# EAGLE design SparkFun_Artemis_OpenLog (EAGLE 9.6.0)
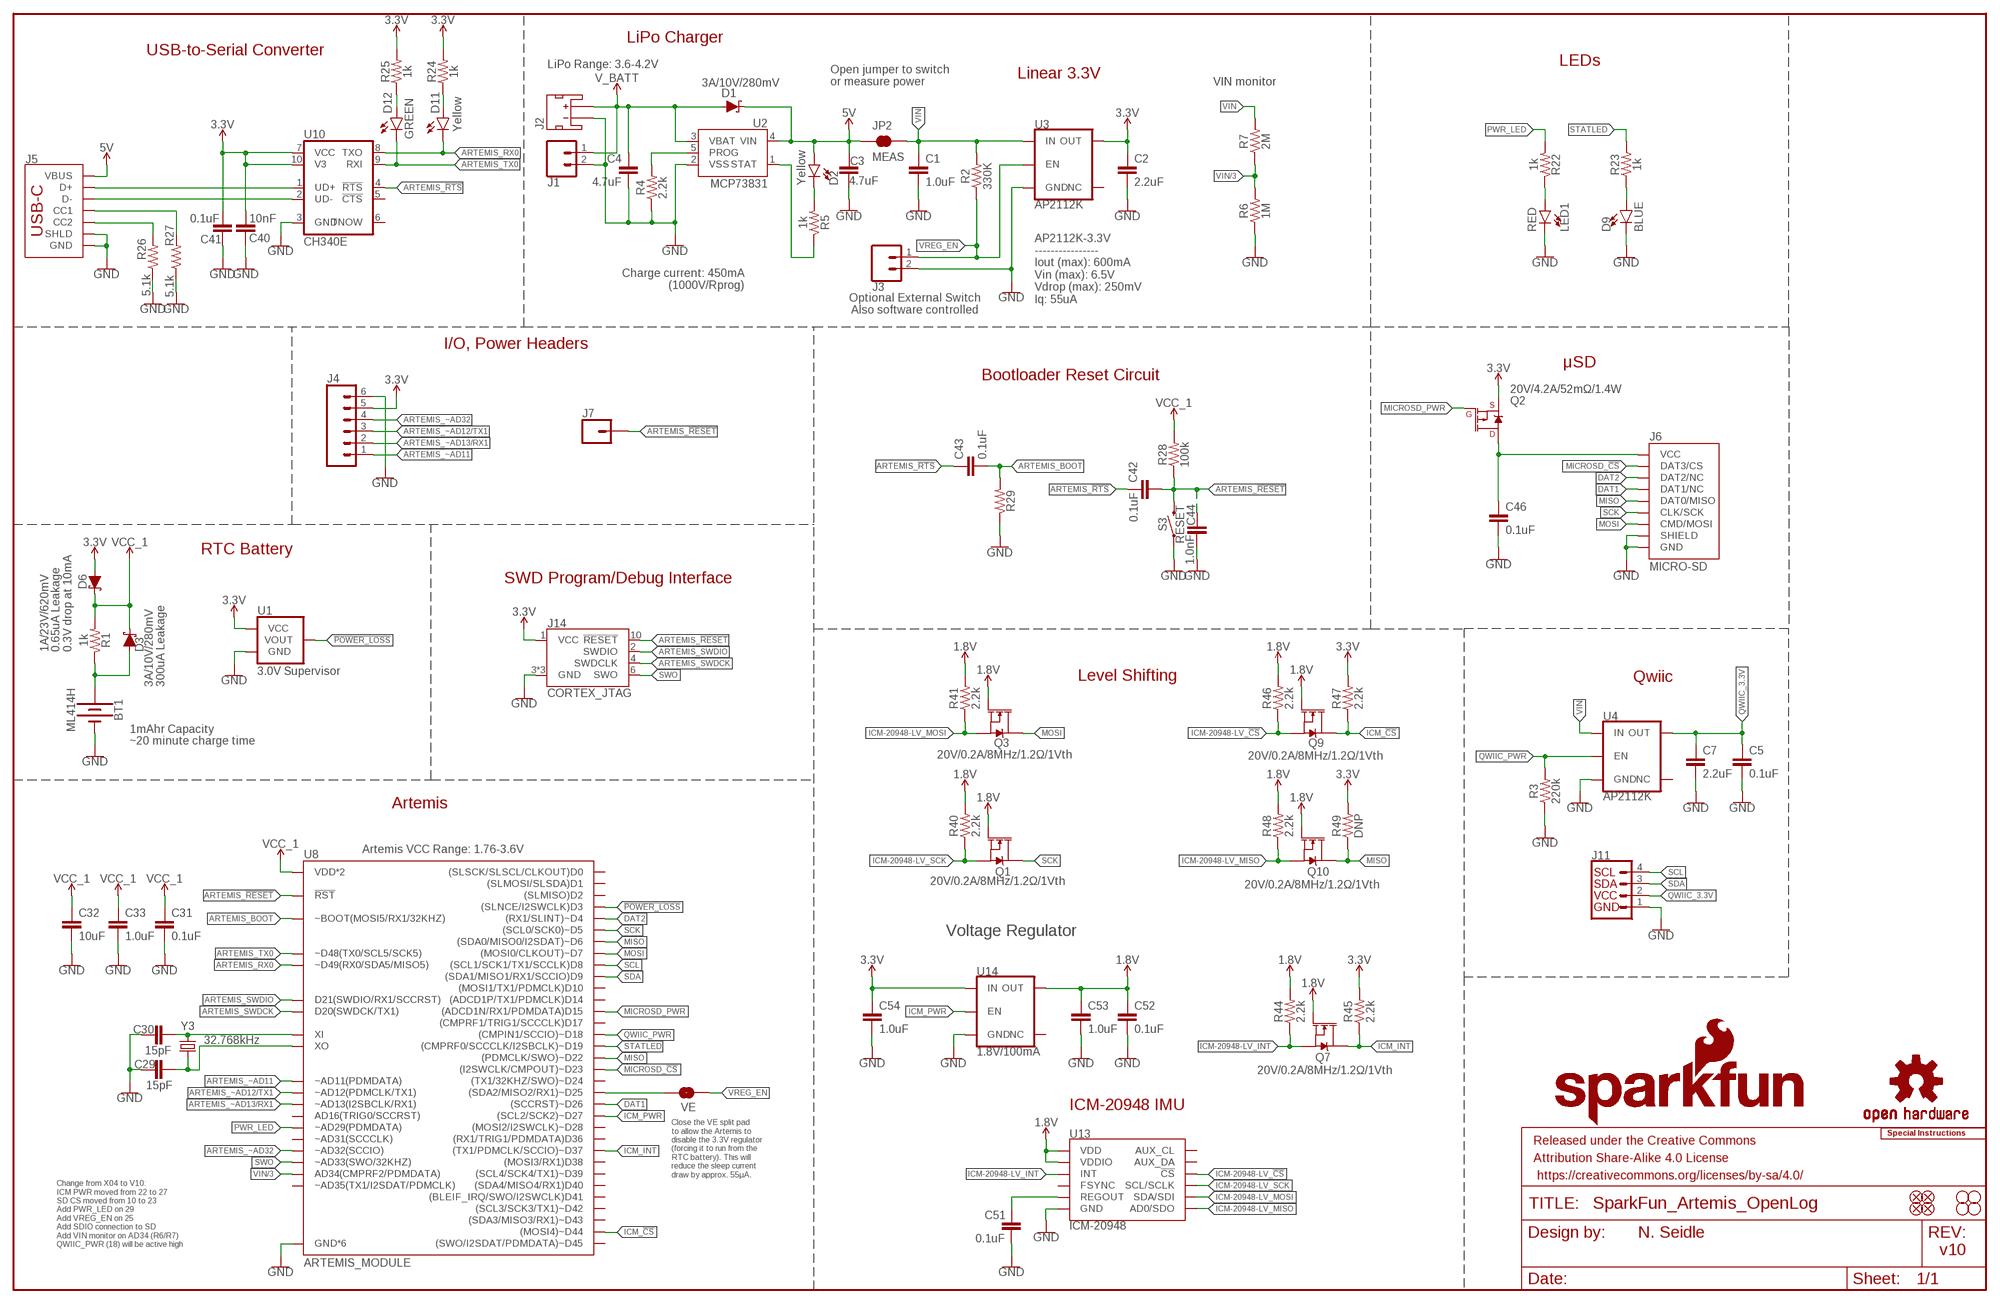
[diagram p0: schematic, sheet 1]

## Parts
BT1  ML414H  ML414H_IV01E_BATTERY  [ML414H_IV01E]
C1  1.0uF  1.0UF-0402T-16V-10%  [0402-TIGHT]
C2  2.2uF  2.2UF-0402_TIGHT-10V-10%-X5R  [0402-TIGHT]
C3  4.7uF  4.7UF-0402_TIGHT-6.3V-20%-X5R  [0402-TIGHT]
C4  4.7uF  4.7UF-0402_TIGHT-6.3V-20%-X5R  [0402-TIGHT]
C5  0.1uF  0.1UF-0402T-6.3V-10%-X7R  [0402-TIGHT]
C7  2.2uF  2.2UF-0402_TIGHT-10V-10%-X5R  [0402-TIGHT]
C29  15pF  15PF-0402T-50V-5%  [0402-TIGHT]
C30  15pF  15PF-0402T-50V-5%  [0402-TIGHT]
C31  0.1uF  0.1UF-0402T-16V-10%  [0402-TIGHT]
C32  10uF  10UF-0402T-6.3V-20%  [0402-TIGHT]
C33  1.0uF  1.0UF-0402T-16V-10%  [0402-TIGHT]
C40  10nF  10NF-0402T-25V-10%  [0402-TIGHT]
C41  0.1uF  0.1UF-0402T-16V-10%  [0402-TIGHT]
C42  0.1uF  0.1UF-0402T-16V-10%  [0402-TIGHT]
C43  0.1uF  0.1UF-0402T-16V-10%  [0402-TIGHT]
C44  1.0nF  1.0NF/1000PF-0402_TIGHT-50V-10%  [0402-TIGHT]
C46  0.1uF  0.1UF-0402T-16V-10%  [0402-TIGHT]
C51  0.1uF  0.1UF-0402T-16V-10%  [0402-TIGHT]
C52  0.1uF  0.1UF-0402T-16V-10%  [0402-TIGHT]
C53  1.0uF  1.0UF-0402T-16V-10%  [0402-TIGHT]
C54  1.0uF  1.0UF-0402T-16V-10%  [0402-TIGHT]
D1  3A/10V/280mV  DIODE-SCHOTTKY-BAT60A  [SOD-323]
D2  Yellow  LED-YELLOW0603  [LED-0603]
D3  3A/10V/280mV  DIODE-SCHOTTKY-BAT60A  [SOD-323]
D6  1A/23V/620mV  DIODE-SCHOTTKY-BAT20J  [SOD-323]
D9  BLUE  LED-BLUE0603  [LED-0603]
D11  Yellow  LED-YELLOW0603  [LED-0603]
D12  GREEN  LED-GREEN0603  [LED-0603]
FD1  FIDUCIAL1X2  [FIDUCIAL-1X2]
FD2  FIDUCIAL1X2  [FIDUCIAL-1X2]
FD3  FIDUCIAL1X2  [FIDUCIAL-1X2]
FD4  FIDUCIAL1X2  [FIDUCIAL-1X2]
FRAME1  FRAME-LEDGER  [CREATIVE_COMMONS]
H1  STAND-OFF  [STAND-OFF]
H2  STAND-OFF  [STAND-OFF]
H3  STAND-OFF  [STAND-OFF]
H4  STAND-OFF  [STAND-OFF]
J1  CONN_021X02_NO_SILK  [1X02_NO_SILK]
J2  JST_2MM_MALE  [JST-2-SMD]
J3  CONN_021X02_NO_SILK  [1X02_NO_SILK]
J4  CONN_06NO_SILK_NO_POP  [1X06_NO_SILK]
J5  USB_C_4-LAYER_PADS  [USB-C-16P_4LAYER-PADS]
J6  MICRO-SD  MICRO-SD-SDIOPUSH-PUSH  [MICRO-SD-SOCKET]
J7  CONN_01PTH_NO_SILK_YES_STOP  [1X01_NO_SILK]
J11  QWIIC_CONNECTORJS-1MM  [JST04_1MM_RA]
J14  CORTEX_JTAG  CORTEX_JTAG_DEBUG_MINIMUM_PTH  [2X5-PTH-1.27MM]
JP2  MEAS  JUMPER-COMBO_2_NC_TRACE  [COMBO-JUMPER_2_NC_TRACE]
LED1  RED  LED-RED0603  [LED-0603]
LOGO1  SFE_LOGO_NAME.1_INCH  [SFE_LOGO_NAME_.1]
LOGO2  OSHW-LOGOS  [OSHW-LOGO-S]
LOGO3  SPECIAL_INSTRUCTIONS-ORDERING  [ORDERING_INSTRUCTIONS]
LOGO4  SFE_LOGO_FLAME.1_INCH  [SFE_LOGO_FLAME_.1]
LOGO5  SFE_LOGO_FLAME.1_INCH  [SFE_LOGO_FLAME_.1]
Q1  20V/0.2A/8MHz/1.2Ω/1Vth  MOSFET-NCH-RE1C00UNTL  [SOT-416FL]
Q2  20V/4.2A/52mΩ/1.4W  MOSFET_PCH-DMG2305UX-7  [SOT23-3]
Q3  20V/0.2A/8MHz/1.2Ω/1Vth  MOSFET-NCH-RE1C00UNTL  [SOT-416FL]
Q7  20V/0.2A/8MHz/1.2Ω/1Vth  MOSFET-NCH-RE1C00UNTL  [SOT-416FL]
Q9  20V/0.2A/8MHz/1.2Ω/1Vth  MOSFET-NCH-RE1C00UNTL  [SOT-416FL]
Q10  20V/0.2A/8MHz/1.2Ω/1Vth  MOSFET-NCH-RE1C00UNTL  [SOT-416FL]
R1  1k  1KOHM-0402T-1/16W-1%  [0402-TIGHT]
R2  330K  330KOHM-0402T-1/16W-1%  [0402-TIGHT]
R3  220k  220KOHM-0402T-1/16W-1%  [0402-TIGHT]
R4  2.2k  2.2KOHM-0402T-1/16W-1%  [0402-TIGHT]
R5  1k  1KOHM-0402T-1/16W-1%  [0402-TIGHT]
R6  1M  1MOHM-0402T-1/16W-1%  [0402-TIGHT]
R7  2M  2MOHM-0402T-1/16W-1%  [0402-TIGHT]
R22  1k  1KOHM-0402T-1/16W-1%  [0402-TIGHT]
R23  1k  1KOHM-0402T-1/16W-1%  [0402-TIGHT]
R24  1k  1KOHM-0402T-1/16W-1%  [0402-TIGHT]
R25  1k  1KOHM-0402T-1/16W-1%  [0402-TIGHT]
R26  5.1k  5.1KOHM-0402T-1/16W-1%  [0402-TIGHT]
R27  5.1k  5.1KOHM-0402T-1/16W-1%  [0402-TIGHT]
R28  100k  100KOHM-0402T-1/16W-1%  [0402-TIGHT]
R29  220KOHM-0402T-1/16W-1%  [0402-TIGHT]
R40  2.2k  2.2KOHM-0402T-1/16W-1%  [0402-TIGHT]
R41  2.2k  2.2KOHM-0402T-1/16W-1%  [0402-TIGHT]
R44  2.2k  2.2KOHM-0402T-1/16W-1%  [0402-TIGHT]
R45  2.2k  2.2KOHM-0402T-1/16W-1%  [0402-TIGHT]
R46  2.2k  2.2KOHM-0402T-1/16W-1%  [0402-TIGHT]
R47  2.2k  2.2KOHM-0402T-1/16W-1%  [0402-TIGHT]
R48  2.2k  2.2KOHM-0402T-1/16W-1%  [0402-TIGHT]
R49  DNP  RESISTOR0402T  [0402-TIGHT]
S3  RESET  MOMENTARY-SWITCH-SPST-SMD-4.6X2.8MM  [TACTILE_SWITCH_SMD_4.6X2.8MM]
U1  3.0V Supervisor  V_SUPERVISOR  [SOT23-3]
U2  MCP73831  [SOT23-5]
U3  AP2112K  V_REG_AP2112K-3.3V  [SOT23-5]
U4  AP2112K  V_REG_AP2112K-3.3V  [SOT23-5]
U8  ARTEMIS_MODULE  ARTEMIS_MODULESMD  [ARTEMIS_FP]
U10  CH340E  CH340E_MSOP10  [MSOP10]
U13  ICM-20948  [QFN24-3X3]
U14  1.8V/100mA  V_REG_SP6214-1.8V  [SC70]
VE  JUMPER-SMT_2_NO_SILK  [SMT-JUMPER_2_NO_SILK]
Y3  32.768kHz  CRYSTAL-32.768KHZSMD-3.2X1.5  [CRYSTAL-SMD-3.2X1.5MM]

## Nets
3.3V: C2.1 C40.1 C41.1 C54.1 D6.A J4.5 J14.1(VCC) Q2.2(S) R24.2 R25.2 R45.2 R47.2 R49.2 U1.3(VCC) U3.5(OUT) U10.7(VCC) U10.10(V3) U14.1(IN)
5V [Power]: C3.1 D1.C D2.A J5.VBUS1(VBUS) J5.VBUS2(VBUS) JP2.1 JP2.3 U2.4(VIN)
!POWER_LOSS!: U1.2(VOUT) U8.D3((SLNCE/I2SWCLK)D3)
ARTEMIS_!RESET: C42.2 C44.1 J7.1 J14.10(!RESET) R28.1 S3.3 S3.4 U8.~RST(!RST)
ARTEMIS_!RTS!: C42.1 C43.1 U10.4(!RTS)
ARTEMIS_BOOT: C43.2 R29.2 U8.BOOT(~BOOT(MOSI5/RX1/32KHZ))
ARTEMIS_RX0: D11.C U8.RXI-0(~D49(RX0/SDA5/MISO5)) U10.8(TXO)
ARTEMIS_SWDCK: J14.4(SWDCLK) U8.SWDCK(D20(SWDCK/TX1))
ARTEMIS_SWDIO: J14.2(SWDIO) U8.SWDIO(D21(SWDIO/RX1/SCCRST))
ARTEMIS_TX0: D12.C U8.TXO-0(~D48(TX0/SCL5/SCK5)) U10.9(RXI)
ARTEMIS_~AD11: J4.1 U8.~AD11(~AD11(PDMDATA))
ARTEMIS_~AD12/TX1: J4.3 U8.~AD12(~AD12(PDMCLK/TX1))
ARTEMIS_~AD13/RX1: J4.2 U8.~AD13(~AD13(I2SBCLK/RX1))
ARTEMIS_~AD32: J4.4 U8.~AD32(~AD32(SCCIO))
CC3: J5.B5(CC2) R26.2
CC4: J5.A5(CC1) R27.2
CHG_LED: R5.1 U2.1(STAT)
D+2: J5.A6(D+) J5.B6(D+) U10.1(UD+)
D-2: J5.A7(D-) J5.B7(D-) U10.2(UD-)
DAT1: J6.RSV2(DAT1/NC) U8.~D26((SCCRST)~D26)
DAT2: J6.RSV1(DAT2/NC) U8.~D4((RX1/SLINT)~D4)
GND: BT1.- C1.2 C2.2 C3.2 C4.2 C5.2 C7.2 C29.1 C30.1 C31.1 C32.2 C33.2 C40.2 C41.2 C44.2 C46.2 C51.2 C52.2 C53.2 C54.2 D9.C J1.2 J2.1(-) J3.2 J4.6 J5.GND J5.GND2(GND) J5.SHLD1(SHLD) J5.SHLD2(SHLD) J5.SHLD3(SHLD) J5.SHLD4(SHLD) J6.CD1(SHIELD) J6.GND J6.GND1(GND) J6.GND3(GND) J11.1 J14.3(GND) J14.5(GND) J14.9(GND) LED1.C R3.1 R4.1 R6.1 R26.1 R27.1 R29.1 S3.1 S3.2 U1.1(GND) U2.2(VSS) U3.2(GND) U4.2(GND) U8.GND@1(GND*6) U8.GND@22(GND*6) U8.GND@38(GND*6) U8.GND@39(GND*6) U8.GND@47(GND*6) U8.GND@59(GND*6) U10.3(GND) U13.18(GND) U13.20(GND) U14.2(GND)
ICM-20948-LV_!CS!: Q9.2(S) R46.1 U13.22(!CS)
ICM-20948-LV_#_1.8V: C52.1 C53.1 Q1.1(G) Q3.1(G) Q7.1(G) Q9.1(G) Q10.1(G) R40.2 R41.2 R44.2 R46.2 R48.2 U13.8(VDDIO) U13.13(VDD) U14.5(OUT) ; supply symbol labelled 1.8V
ICM-20948-LV_INT: Q7.2(S) R44.1 U13.12(INT)
ICM-20948-LV_MISO: Q10.2(S) R48.1 U13.9(AD0/SDO)
ICM-20948-LV_MOSI: Q3.2(S) R41.1 U13.24(SDA/SDI)
ICM-20948-LV_SCK: Q1.2(S) R40.1 U13.23(SCL/SCLK)
ICM_!CS!: Q9.3(D) R47.1 U8.~D44((MOSI4)~D44)
ICM_INT: Q7.3(D) R45.1 U8.~D37((TX1/PDMCLK/SCCIO)~D37)
ICM_PWR: U8.~D27((SCL2/SCK2)~D27) U14.3(EN)
MICROSD_!CS!: J6.CS(DAT3/CS) U8.~D23((I2SWCLK/CMPOUT)~D23)
MICROSD_PWR: Q2.1(G) U8.D15((ADCD1N/RX1/PDMDATA)D15)
MISO: J6.DO(DAT0/MISO) Q10.3(D) R49.1 U8.~D6((SDA0/MISO0/I2SDAT)~D6) U8.~D22((PDMCLK/SWO)~D22)
MOSI: J6.DI(CMD/MOSI) Q3.3(D) U8.D7((MOSI0/CLKOUT)~D7)
N$1: BT1.+ D3.A R1.1
N$7: R4.2 U2.5(PROG)
N$11: D2.C R5.2
N$20: C29.2 U8.XO Y3.P$2
N$21: C30.2 U8.XI Y3.P$1
N$24: LED1.A R22.1
N$25: D9.A R23.1
N$26: D12.A R25.1
N$27: D11.A R24.1
N$30: C51.1 U13.10(REGOUT)
PWR_LED: R22.2 U8.~AD29(~AD29(PDMDATA))
QWIIC_3.3V: C5.1 C7.1 J11.2 U4.5(OUT)
QWIIC_PWR: R3.2 U4.3(EN) U8.~D18((CMPIN1/SCCIO)~D18)
SCK: J6.SCLK(CLK/SCK) Q1.3(D) U8.~D5((SCL0/SCK0)~D5)
SCL: J11.4 U8.D8((SCL1/SCK1/TX1/SCCLK)D8)
SD_PWR: C46.1 J6.VCC Q2.3(D)
SDA: J11.3 U8.D9((SDA1/MISO1/RX1/SCCIO)D9)
STATLED: R23.2 U8.~D19((CMPRF0/SCCCLK/I2SBCLK)~D19)
SWO: J14.6(SWO) U8.~AD33/SWO(~AD33(SWO/32KHZ))
V_BATT: C4.1 D1.A J1.1 J2.2(+) U2.3(VBAT)
VCC_1: C31.2 C32.1 C33.1 D3.C D6.C R1.2 R28.2 U8.VDD@36(VDD*2) U8.VDD@37(VDD*2)
VIN [Power]: C1.1 JP2.2 JP2.4 R2.2 R7.2 U3.1(IN) U4.1(IN)
VIN/3: R6.2 R7.1 U8.AD34(AD34(CMPRF2/PDMDATA))
VREG_EN: J3.1 R2.1 U3.3(EN) VE.2
VREG_EN1: U8.~D25((SDA2/MISO2/RX1)~D25) VE.1
Unconnected: J2.NC1(PAD1) J2.NC2(PAD2) U3.4(NC) U4.4(NC) U8.AD16(AD16(TRIG0/SCCRST)) U8.D0((SLSCK/SLSCL/CLKOUT)D0) U8.D1((SLMOSI/SLSDA)D1) U8.D2((SLMISO)D2) U8.D10((MOSI1/TX1/PDMCLK)D10) U8.D14((ADCD1P/TX1/PDMCLK)D14) U8.D17((CMPRF1/TRIG1/SCCCLK)D17) U8.D36((RX1/TRIG1/PDMDATA)D36) U8.D38((MOSI3/RX1)D38) U8.D40((SDA4/MISO4/RX1)D40) U8.D41((BLEIF_IRQ/SWO/I2SWCLK)D41) U8.~AD31(~AD31(SCCCLK)) U8.~AD35(~AD35(TX1/I2SDAT/PDMCLK)) U8.~D24((TX1/32KHZ/SWO)~D24) U8.~D28((MOSI2/I2SWCLK)~D28) U8.~D39((SCL4/SCK4/TX1)~D39) U8.~D42((SCL3/SCK3/TX1)~D42) U8.~D43((SDA3/MISO3/RX1)~D43) U8.~D45((SWO/I2SDAT/PDMDATA)~D45) U10.5(!CTS) U10.6(TNOW) U13.7(AUX_CL) U13.11(FSYNC) U13.21(AUX_DA) U14.4(NC)

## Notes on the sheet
- LiPo Charger
- USB-to-Serial Converter
- LiPo Range: 3.6-4.2V | LEDs
- Linear 3.3V
- Open jumper to switch
  or measure power
- VIN monitor
- AP2112K-3.3V
  ----------------
  Iout (max): 600mA 
  Vin (max): 6.5V
  Vdrop (max): 250mV
  Iq: 55uA
- Charge current: 450mA
  (1000V/Rprog)
- Optional External Switch
  Also software controlled
- I/O, Power Headers
- μSD
- Bootloader Reset Circuit
- RTC Battery
- SWD Program/Debug Interface
- 0.65uA Leakage
  0.3V drop at 10mA
- Level Shifting | Qwiic
- 300uA Leakage
- 1mAhr Capacity
- ~20 minute charge time
- Artemis
- Artemis VCC Range: 1.76-3.6V
- Voltage Regulator
- ICM-20948 IMU
- Close the VE split pad
  to allow the Artemis to
  disable the 3.3V regulator
  (forcing it to run from the
  RTC battery). This will
  reduce the sleep current
  draw by approx. 55μA.
- N. Seidle
- Change from X04 to V10:
  ICM PWR moved from 22 to 27
  SD CS moved from 10 to 23
  Add PWR_LED on 29
  Add VREG_EN on 25
  Add SDIO connection to SD
  Add VIN monitor on AD34 (R6/R7)
  QWIIC_PWR (18) will be active high
- v10

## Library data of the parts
BT1 = SparkFun-Batteries:ML414H_IV01E_BATTERY: SEIKO ML414H-IV01E Reflowable Lithium Battery; PROD_ID: BATT-14267
C1 C33 C53 C54 = SparkFun-Capacitors:1.0UF: 1µF ceramic capacitors; PROD_ID: CAP-12417
C2 C7 = SparkFun-Capacitors:2.2UF: 2.2µF ceramic capacitors; PROD_ID: CAP-14232
C3 C4 = SparkFun-Capacitors:4.7UF: 4.7µF ceramic capacitors; PROD_ID: CAP-14240
C5 = SparkFun-Capacitors:0.1UF: 0.1µF ceramic capacitors; PROD_ID: CAP-14993
C29 C30 = SparkFun-Capacitors:15PF: 15pF ceramic capacitors; PROD_ID: CAP-13063
C31 C41-C43 C46 C51 C52 = SparkFun-Capacitors:0.1UF: 0.1µF ceramic capacitors; PROD_ID: CAP-12416
C32 = SparkFun-Capacitors:10UF: 10.0µF ceramic capacitors; PROD_ID: CAP-14848
C40 = SparkFun-Capacitors:10NF: 0.01uF/10nF/10,000pF ceramic capacitors; PROD_ID: CAP-14847
C44 = SparkFun-Capacitors:1.0NF/1000PF: 1nF/1,000pF ceramic capacitors; PROD_ID: CAP-14280
D1 D3 = SparkFun-DiscreteSemi:DIODE-SCHOTTKY: Schottky diode; PROD_ID: DIO-14072
D2 D11 = SparkFun-LED:LED-YELLOW: Yellow SMD LED; PROD_ID: DIO-09003
D6 = SparkFun-DiscreteSemi:DIODE-SCHOTTKY: Schottky diode; PROD_ID: DIO-11623
D9 = SparkFun-LED:LED-BLUE: Blue SMD LED; PROD_ID: DIO-08575
D12 = SparkFun-LED:LED-GREEN: Green SMD LED; PROD_ID: DIO-00821
FD1-FD4 = SparkFun-Aesthetics:FIDUCIAL: Fiducial Alignment Points
FRAME1 = SparkFun-Aesthetics:FRAME-LEDGER: Schematic Frame - Ledger
H1-H4 = SparkFun-Hardware:STAND-OFF: Stand Off
J1 J3 = SparkFun-Connectors:CONN_02: Multi connection point. Often used as Generic Header-pin footprint for 0.1 inch spaced/style header connections
J2 = SparkFun-Connectors:JST_2MM_MALE: JST 2MM MALE RA CONNECTOR Two pin, compact surface mount connector. Commonly used as a battery input connection point. We really like the solid locking feeling and high current rating on these small connectors. We use these all the time as battery connectors. Mates to single-cell LiPo batteries.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; PROD_ID: CONN-11443; SF_ID: PRT-08612
J4 = SparkFun-Connectors:CONN_06: Multi connection point. Often used as Generic Header-pin footprint for 0.1 inch spaced/style header connections On any of the 0.1 inch spaced packages, you can populate with these: Break Away Headers - Straight (PRT-00116) Break Away Male Headers - Right Angle (PRT-00553) Female Headers (PRT-00115)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
J5 = SparkFun-Connectors:USB_C: USB Type C 16Pin Connector Super Speed pins not available on the 16-pin purely SMD connector so this part is best for USB 2.0 implementations. D1 and D2 are tied together enabling D+/- no matter which way the cable is plugged into the connector. The two channel configuration pins (CC1/2) are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; PROD_ID: CONN-14122
J6 = SparkFun-Connectors:MICRO-SD-SDIO: microSD Socket for Transflash Push-push type µSD socket. tDoc lines correctly indicate media card edge positions when inserting (unlocked, locked, depressed). NOTE: CD1 and CD2 are connected internally, and the default detect state of the socket is detect pin to ground. SparkFun Products: WAV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; PROD_ID: CONN-07820
J7 = SparkFun-Connectors:CONN_01: Single connection point. Often used as Generic Header-pin footprint for 0.1 inch spaced/style header connections
J11 = SparkFun-Connectors:QWIIC_CONNECTOR: SparkFun I2C Standard Qwiic Connector An SMD 1mm pitch JST connector makes it easy and quick (get it? Qwiic?) to connect I2C devices to each other. The Qwiic system enables fast and solderless connection between popular platforms and various sensors and actuators. We carry 200mm, 100mm, 50mm, and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; PROD_ID: CONN-13694; VALUE: QWIIC_RIGHT_ANGLE
J14 = SparkFun-Connectors:CORTEX_JTAG_DEBUG_MINIMUM: Cortex Debug Connector - 10 pin Supports JTAG debug, Serial Wire debug, and Serial Wire Viewer. PTH and SMD connector options available. General Connector Information Products: PTH Connector -via Digi-Key SparkFun PSoc SparkFun T
JP2 = SparkFun-Jumpers:JUMPER-COMBO_2_NC_TRACE
LED1 = SparkFun-LED:LED-RED: Red SMD LED; PROD_ID: DIO-00819
LOGO1 = SparkFun-Aesthetics:SFE_LOGO_NAME: SparkFun Font Logo
LOGO2 = SparkFun-Aesthetics:OSHW-LOGO: Open-Source Hardware (OSHW) Logo
LOGO3 = SparkFun-Aesthetics:SPECIAL_INSTRUCTIONS: Special Ordering/Production Instructions Alert
LOGO4 LOGO5 = SparkFun-Aesthetics:SFE_LOGO_FLAME: SparkFun Flame Logo
Q1 Q3 Q7 Q9 Q10 = SparkFun-DiscreteSemi:MOSFET-NCH: N-channel MOSFETs Voltage controlled devices that allow control of high current outputs. SparkFun Products: SparkFun OpenScale SparkFun Digital Sandbox SparkFun Monster Moto Shield SparkFun MOSFET Power Controller; PROD_ID: TRANS-14399
Q2 = SparkFun-DiscreteSemi:MOSFET_PCH: P-channel MOSFETs Voltage controlled devices that allow control of high current outputs. SparkFun Products: SparkFun ESP32 Thing SparkFun ESP8266 Thing SparkFun Pi Servo HAT V2 DMG2305UX-7 (20V/4.2A/SOT23-3); PROD_ID: TRAN-14388
R1 R5 R22-R25 = SparkFun-Resistors:1KOHM: 1kΩ resistor; PROD_ID: RES-14342
R2 = New_Parts:330KOHM: 330kΩ resistor
R3 R29 = SparkFun-Resistors:220KOHM: 220kΩ resistor; PROD_ID: RES-15094
R4 R40 R41 R44-R48 = SparkFun-Resistors:2.2KOHM: 2.2kΩ resistor; PROD_ID: RES-14341
R6 = New_Parts:1MOHM: 1MΩ resistor
R7 = New_Parts:2MOHM: 2MΩ resistor
R26 R27 = SparkFun-Resistors:5.1KOHM; PROD_ID: RES-14340
R28 = SparkFun-Resistors:100KOHM: 100kΩ resistor; PROD_ID: RES-13495
R49 = SparkFun-Resistors:RESISTOR: Generic Resistor Package
S3 = SparkFun-Switches:MOMENTARY-SWITCH-SPST: Momentary Switch (Pushbutton) - SPST; PROD_ID: SWCH-13065
U1 = SparkFun-IC-Power:V_SUPERVISOR: BD48xxx - Voltage Detector IC ROHM’s BD48xxx and BD49xxx series are highly accurate, low-current Voltage Detector IC series. The family includes BD48xxx devices with N-channel open drain output and BD49xxx devices with CMOS output. The devices are available for specific detection voltages ranging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; PROD_ID: IC-14809
U2 = SparkFun-IC-Power:MCP73831: MCP73831T Li-Ion, Li-Pol Controller Miniature single cell, fully integrated Li-Ion, Li-polymer charge management controller Datasheet SparkFun Products: SparkFun ESP32 Thing SparkFun 9DoF Razor IMU M0; PROD_ID: IC-09995
U3 U4 = SparkFun-IC-Power:V_REG_AP2112: AP2112 - 600mA CMOS LDO Regulator w/ Enable The AP2112 is CMOS process low dropout linear regulator with enable function, the regulator delivers a guaranteed 600mA (min.) continuous load current. Features Output Voltage Accuracy: ±1.5% Output Current: 600mA (Min.) Foldback Short Current Protection: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; PROD_ID: VREG-12457; VALUE: 3.3V
U8 = SparkFun-IC-Microcontroller:ARTEMIS_MODULE: Description: The Artemis Module from SparkFun is a Cortex-M4F with BLE 5.0 running up to 96MHz and with as low power as 6uA per MHz (less than 5mW). This is the world's first module to bridge the market between hobbyists and consumer products. We've packaged all the power of a modern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; PROD_ID: SUB-14479
U10 = SparkFun-IC-Comms:CH340E; PROD_ID: IC-14135
U13 = SparkFun-Sensors:ICM-20948: ICM-20948 9 Degree of Freedom IMU World’s lowest power 9-axis MotionTracking device that is ideally suited for smartphones, tablets, wearable sensors, and IoT applications. Includes onboard Digital Motion Processor to offload computations from the host processor Datasheet SparkFun Products: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; PROD_ID: IC-14247; VALUE: 9DoF IMU
U14 = SparkFun-IC-Power:V_REG_SP6214: Voltage Regulator - SP6214 SP6214 Series SC-70-5 Micropower SC-70 100 mA CMOS LDO Regulator Datasheet SparkFun Products: MP3 Trigger SparkFun Particle Sensor Breakout; PROD_ID: VREG-08428
VE = SparkFun-Jumpers:JUMPER-SMT_2_NO: Normally open jumper
Y3 = SparkFun-Clocks:CRYSTAL-32.768KHZ: 32.768kHz Crystal; PROD_ID: XTAL-13062

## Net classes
1 Power: width 0.457 mm

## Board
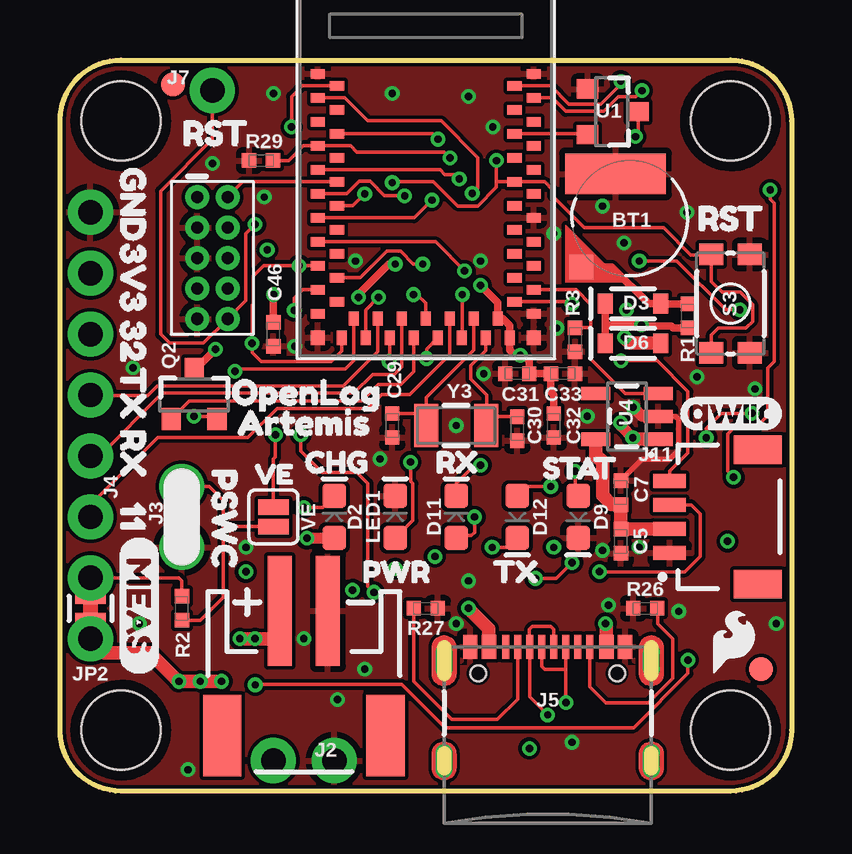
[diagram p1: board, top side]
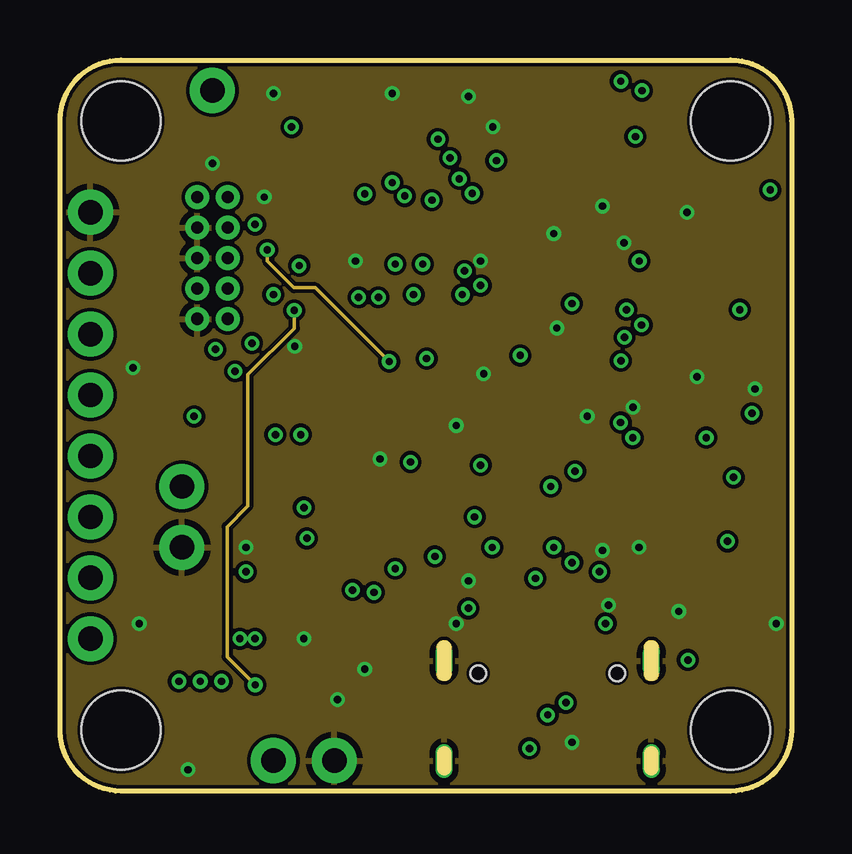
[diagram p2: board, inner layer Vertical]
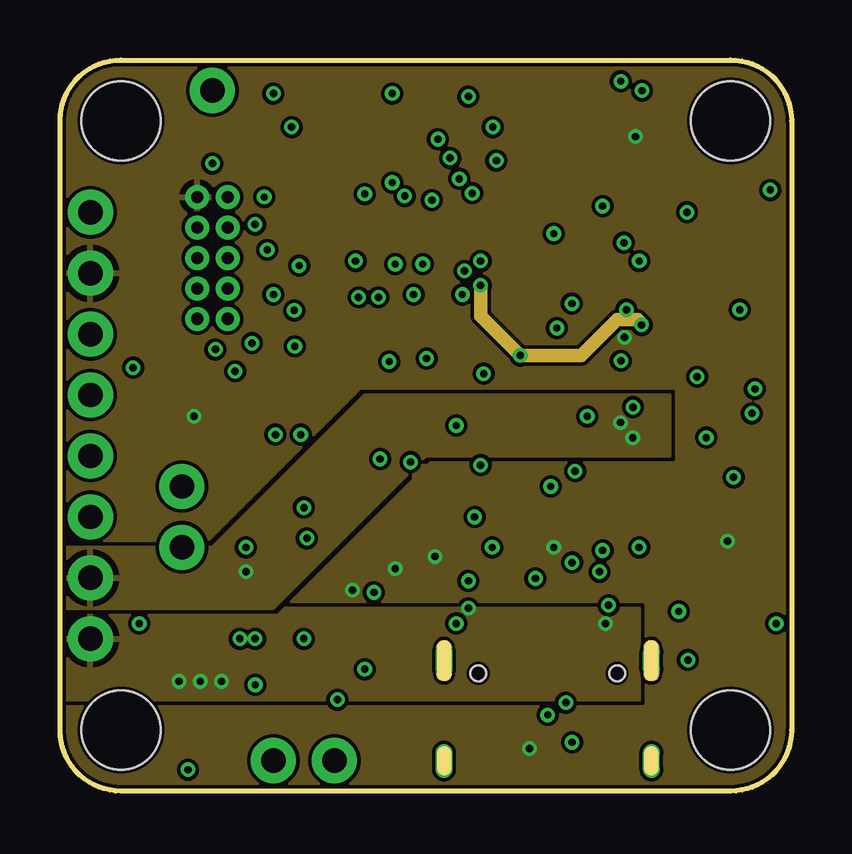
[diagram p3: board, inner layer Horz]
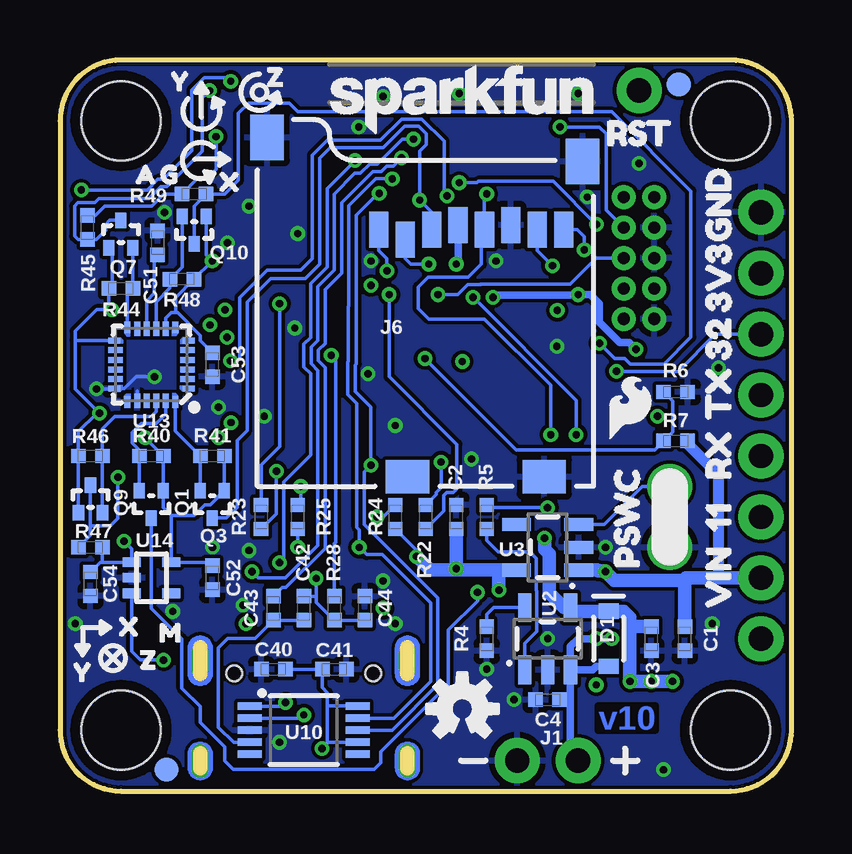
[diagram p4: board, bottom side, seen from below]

Size 30.48 x 30.48 mm. Coordinates in mm from the lower left corner, seen from the top.
Outline: 27.94,0 2.54,0 arc-90 0,2.54 0,27.94 arc-90 2.54,30.48 27.94,30.48 arc-90 30.48,27.94 30.48,2.54 arc-90 27.94,0
Copper layers (1+2*15+16): Top 0.035mm / dielectric 1.5mm / Vertical 0.035mm / dielectric 0.15mm / Horz 0.035mm / dielectric 0.2mm / Bottom 0.035mm
Design rules "SparkFun-2-layer-PCBWay-LIMIT *": minimum track width 6mil, minimum drill 0.3mm, track to track 6mil, track to pad 6mil, pad to pad 6mil, via to via 6mil, smd to smd 6mil, copper to edge 6mil, drill to drill 6mil, minimum pad ring 6mil, minimum via ring 6mil, stop-mask expansion 4mil, vias tented up to drill 25mil, thermal gap 10mil

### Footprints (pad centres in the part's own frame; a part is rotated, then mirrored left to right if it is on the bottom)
ML414H_IV01E = smd 1 x 1: + 2.022,2.032 | smd 4.2 x 1.7: - 0.6,-1.85
0402-TIGHT = smd 0.6 x 0.6: 1 -0.5,0; 2 0.5,0
SOD-323 = smd 0.63 x 0.83: A 1.15,0; C -1.15,0
LED-0603 = smd 1 x 1: A -0.877,0; C 0.877,0
FIDUCIAL-1X2 = smd 1 x 1: 1 0,0
STAND-OFF = hole 3.302: 0,0
1X02_NO_SILK = drill 1.016 pad 1.88: 1 0,0; 2 2.54,0
JST-2-SMD = smd 1 x 4.6: 1 -1,-3.7; 2 1,-3.7 | smd 1.6 x 3.4: NC1 -3.4,1.5; NC2 3.4,1.5
1X06_NO_SILK = drill 1.016 pad 1.88: 1 0,0; 2 2.54,0; 3 5.08,0; 4 7.62,0; 5 10.16,0; 6 12.7,0
USB-C-16P_4LAYER-PADS = smd 0.3 x 1: A5 -1.25,-0.34; A6 -0.25,-0.34; A7 0.25,-0.34; A8 1.25,-0.34; B5 1.75,-0.34; B6 0.75,-0.34; B7 -0.75,-0.34; B8 -1.75,-0.34 | smd 0.6 x 1: GND -3.225,-0.34; GND2 3.225,-0.34; VBUS1 -2.45,-0.34; VBUS2 2.45,-0.34 | drill 0.4 pad 0.6 long: SHLD1 -4.318,-0.915; SHLD2 4.318,-0.915; SHLD3 -4.318,-5.095; SHLD4 4.318,-5.095 | hole 0.65: -2.89,-1.445; 2.89,-1.445
MICRO-SD-SOCKET = smd 1.8 x 1.4: CD1 -2.05,0.4; CD2 -7.75,0.4 | smd 0.8 x 1.5: CS -7.84,10.3; DI -6.74,10.7; DO -2.34,10.7; GND -3.44,10.9; RSV1 -8.94,10.7; RSV2 -1.24,10.7; SCLK -4.54,10.7; VCC -5.64,10.9 | smd 1.4 x 1.9: GND1 -13.6,14.55; GND3 -0.45,13.55
1X01_NO_SILK = drill 1.016 pad 1.88: 1 0,0
JST04_1MM_RA = smd 0.6 x 1.35: 1 -1.5,0; 2 -0.5,0; 3 0.5,0; 4 1.5,0 | smd 1.2 x 2: NC1 2.8,-3.675; NC2 -2.8,-3.675
2X5-PTH-1.27MM = drill 0.508 pad 1: 1 -2.54,-0.635; 2 -2.54,0.635; 3 -1.27,-0.635; 4 -1.27,0.635; 5 0,-0.635; 6 0,0.635; 7 1.27,-0.635; 8 1.27,0.635; 9 2.54,-0.635; 10 2.54,0.635
COMBO-JUMPER_2_NC_TRACE = smd 0.635 x 1.27: 1 -0.508,0; 2 0.508,0 | drill 1.016 pad 1.88: 3 -1.27,0; 4 1.27,0
SOT-416FL = smd 0.46 x 0.65: 1 -0.5,-1.1; 2 0.5,-1.1; 3 0,0.05
SOT23-3 = smd 0.8 x 0.9: 1 -0.95,-1; 2 0.95,-1; 3 0,1.1
TACTILE_SWITCH_SMD_4.6X2.8MM = smd 0.9 x 1: 1 -2.05,-0.8; 2 2.05,-0.8; 3 2.05,0.8; 4 -2.05,0.8
SOT23-5 = smd 0.55 x 1.2: 1 -0.95,-1.3; 2 0,-1.3; 3 0.95,-1.3; 4 0.95,1.3; 5 -0.95,1.3
ARTEMIS_FP = smd 0.4 x 0.6: AD16 -4,-3.7; BOOT 1.5,4.5; D0 0.5,-4.5; D1 -0.5,-4.5; D2 -1,-3.7; D3 2,-3.7; D7 -1.5,4.5; D8 -0.5,4.5; D9 2,3.7; D10 1,3.7; D14 -5,3.7; D17 -3.5,-4.5; D36 2.5,-4.5; D38 3,-3.7; D40 2.5,4.5; D41 -2.5,-4.5; GND@1 4.5,4.5; GND@39 -5.5,-4.5; GND@47 -1.5,-4.5; GND@59 4.5,-4.5; RXI-0 3.5,4.5; SWDCK 4,3.7; SWDIO 0,3.7; TXO-0 0.5,4.5; ~AD31 -3,-3.7; ~AD35 -2,3.7; ~D4 -2.5,4.5; ~D5 -1,3.7; ~D18 -4.5,-4.5; ~D19 -5,-3.7; ~D22 -3.5,4.5; ~D23 -4,3.7; ~D24 -3,3.7; ~D27 -4.5,4.5; ~D28 -5.5,4.5; ~D37 3.5,-4.5; ~D39 3,3.7; ~D42 1.5,-4.5; ~D43 1,-3.7; ~D44 4,-3.7; ~D45 -2,-3.7; ~RST 0,-3.7 | smd 0.6 x 0.4: AD34 -6.5,-0.5; D15 -6.5,0.5; VDD@36 -5.7,-3; VDD@37 -6.5,-3.5; XI -6.5,-2.5; XO -5.7,-2; ~AD11 -5.7,-1; ~AD12 -5.7,2; ~AD13 -5.7,1; ~AD29 -6.5,-1.5; ~AD32 -5.7,3; ~AD33/SWO -5.7,0; ~D6 -6.5,3.5; ~D25 -6.5,2.5; ~D26 -6.5,1.5 | smd 0.6 x 0.6: GND@22 -6.5,4.5; GND@38 -6.5,-4.5
MSOP10 = smd 1 x 0.3: 1 -2.25,1; 2 -2.25,0.5; 3 -2.25,0; 4 -2.25,-0.5; 5 -2.25,-1; 6 2.25,-1; 7 2.25,-0.5; 8 2.25,0; 9 2.25,0.5; 10 2.25,1
QFN24-3X3 = smd 0.495 x 0.25: 1 -1.552,1; 6 -1.552,-1; 13 1.552,-1; 18 1.552,1 | smd 0.6 x 0.25: 2 -1.5,0.6; 3 -1.5,0.2; 4 -1.5,-0.2; 5 -1.5,-0.6; 14 1.5,-0.6; 15 1.5,-0.2; 16 1.5,0.2; 17 1.5,0.6 | smd 0.25 x 0.495: 7 -1,-1.552; 12 1,-1.552; 19 1,1.552; 24 -1,1.552 | smd 0.25 x 0.6: 8 -0.6,-1.5; 9 -0.2,-1.5; 10 0.2,-1.5; 11 0.6,-1.5; 20 0.6,1.5; 21 0.2,1.5; 22 -0.2,1.5; 23 -0.6,1.5
SC70 = smd 0.4 x 0.75: 1 -0.65,-0.825; 2 0,-0.825; 3 0.65,-0.825; 4 0.65,0.825; 5 -0.65,0.825
SMT-JUMPER_2_NO_SILK = smd 0.635 x 1.27: 1 -0.406,0; 2 0.406,0
CRYSTAL-SMD-3.2X1.5MM = smd 1 x 1.8: P$1 -1.25,0; P$2 1.25,0

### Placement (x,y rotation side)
BT1  23.75,23.88 180 top
C1  4.45,6.35 270 bottom
C2  13.97,11.43 90 bottom
C3  5.84,6.35 270 bottom
C4  10.16,3.81 180 bottom
C5  23.37,10.41 270 top
C7  23.37,12.45 90 top
C29  13.84,15.24 90 top
C30  19.05,15.11 90 top
C31  19.05,17.4 0 top
C32  20.57,15.24 270 top
C33  20.95,17.4 0 top
C40  21.59,5.08 180 bottom
C41  19.05,5.08 0 bottom
C42  20.32,7.62 90 bottom
C43  21.59,7.62 90 bottom
C44  17.78,7.62 90 bottom
C46  8.89,19.05 270 top
C51  26.42,22.86 90 bottom
C52  24.13,8.89 270 bottom
C53  24.13,17.78 270 bottom
C54  29.21,8.64 270 bottom
D1  7.62,6.35 270 bottom
D2  11.43,11.43 90 top
D3  23.88,20.32 0 top
D6  23.88,18.67 0 top
D9  21.59,11.43 270 top
D11  16.51,11.43 90 top
D12  19.05,11.43 270 top
FD1  29.21,5.08 0 top
FD2  4.7,29.46 0 bottom
FD3  4.7,29.46 0 top
FD4  26.04,0.89 0 bottom
FRAME1  not placed on the board
H1  2.54,2.54 0 bottom
H2  27.94,2.54 0 bottom
H3  2.54,27.94 0 bottom
H4  27.94,27.94 0 bottom
J1  8.89,1.27 180 bottom
J2  10.16,3.81 180 top
J3  5.08,12.7 270 top
J4  1.27,11.43 90 top
J5  20.32,6.35 0 top
J6  8.26,12.7 0 bottom
J7  6.35,29.21 0 top
J11  25.4,11.43 90 top
J14  6.35,22.23 270 top
JP2  1.27,7.62 90 top
LED1  13.97,11.43 90 top
LOGO1  13.72,28.83 0 bottom
LOGO2  13.72,3.43 0 bottom
LOGO3  not placed on the board
LOGO4  28.07,6.22 0 top
LOGO5  6.73,16 0 bottom
Q1  26.67,11.43 180 bottom
Q2  5.59,16.51 0 top
Q3  24.13,11.43 180 bottom
Q7  27.94,23.75 0 bottom
Q9  29.21,12.7 0 bottom
Q10  24.89,22.86 180 bottom
R1  26.16,19.81 270 top
R2  5.08,7.62 90 top
R3  21.46,18.82 90 top
R4  12.7,6.35 90 bottom
R5  12.7,11.43 90 bottom
R6  4.83,16.64 180 bottom
R7  4.83,14.61 0 bottom
R22  15.24,11.43 270 bottom
R23  22.1,11.43 90 bottom
R24  16.51,11.43 270 bottom
R25  20.57,11.43 270 bottom
R26  24.38,7.62 0 top
R27  15.24,7.62 180 top
R28  19.05,7.62 90 bottom
R29  8.38,26.29 0 top
R40  26.67,13.97 0 bottom
R41  24.13,13.97 0 bottom
R44  27.94,20.95 180 bottom
R45  29.34,23.5 90 bottom
R46  29.21,13.97 180 bottom
R47  29.21,10.16 0 bottom
R48  25.4,21.34 0 bottom
R49  24.89,24.89 180 bottom
S3  27.94,20.32 90 top
U1  22.99,28.32 270 top
U2  10.16,6.35 0 bottom
U3  10.16,10.16 90 bottom
U4  23.62,15.62 90 top
U8  15.24,25.4 90 top
U10  20.32,2.54 0 bottom
U13  26.67,17.78 180 bottom
U14  26.67,8.89 270 bottom
U$1  [QWIIC#LOGO#JPG]  27.94,15.75 0 top
U$2  [CHG2]  9.4,13.72 0 top
U$3  [PWR0]  11.81,9.14 0 top
U$4  [RX4]  14.86,13.72 0 top
U$5  [STAT5]  19.3,13.46 0 top
U$6  [VE0]  7.37,13.21 0 top
U$7  [TX3]  17.27,9.14 0 top
U$8  [RST0]  4.19,27.43 0 top
U$9  [ARTEMIS13]  6.48,15.37 0 top
U$10  [PSWC0]  6.86,8.38 90 bottom
U$11  [PSWC0]  6.86,14.35 270 top
U$12  [RST0]  8.64,27.43 0 bottom
U$27  [MEAS3]  3.3,10.67 270 top
U$28  [OPENLOG12]  6.22,16.64 0 top
U$32  [RST9]  25.65,23.88 0 top
U$33  [VIN8]  3.05,6.73 90 bottom
U$34  [3V34]  3.05,23.75 270 top
U$35  [3V34]  3.05,19.05 90 bottom
U$36  [113]  3.05,12.95 270 top
U$37  [113]  3.05,9.91 90 bottom
U$38  [322]  3.05,20.7 270 top
U$39  [322]  3.05,16.89 90 bottom
U$40  [GND5]  3.05,27.05 270 top
U$41  [GND5]  3.05,21.84 90 bottom
U$42  [RX1]  3.05,16 270 top
U$43  [X0]  24.51,25.4 0 bottom
U$44  [Y1]  26.54,29.59 0 bottom
U$45  [Z2]  22.56,29.77 0 bottom
U$46  [G5]  27,25.7 0 bottom
U$47  [A4]  28.02,25.7 0 bottom
U$48  [M3]  27.05,6.6 0 bottom
U$49  [X0]  28.7,6.86 0 bottom
U$50  [Y1]  30.61,4.95 0 bottom
U$51  [Z2]  25.78,5.46 180 bottom
U$54  [RX1]  3.05,12.06 90 bottom
U$55  [TX0]  3.05,18.54 270 top
U$56  [TX0]  3.05,14.61 90 bottom
VE  8.89,11.43 270 top
Y3  16.51,15.24 180 top

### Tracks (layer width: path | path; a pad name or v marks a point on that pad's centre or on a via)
3.3V  (via drill 0.3)
  Top 0.152: U1.3 24.09,27.39 v23.98,27.29 | Q2.2 6.43,15.62 v5.59,15.62
  Top 0.559: D6.A 23.77,18.67 v23.52,18.92
  Bottom 0.152: 19.34,1.99 19.34,3.56 | U10.10 18.09,3.56 19.34,3.56 | U3.5 11.56,9.31 | v27.81,10.41 27.5,10.1 U14.1 28.7,9.54 | R45.2 29,24 28.61,24.38 26.66,24.38 26.15,24.89 R49.2 24.76,25.53 24.38,25.53 23.98,25.93 v23.98,27.29 | R24.2 15.62,10.03 v15.62,9.78 | R25.2 v20.57,10.16 | 19.34,1.99 v19.56,1.78 | 19.34,1.99 19.3,2.04 U10.7 | 19.34,3.56 19.34,4.1 19.56,4.32 C41.1 C40.1 | C54.1 28.81,9.54 28.7,9.54 | R47.2 28.71,9.55 28.7,9.54
  Bottom 0.559: U3.5 12.19,9.21 | v12.19,8.38 12.19,9.21 | 12.19,9.21 13.97,9.21 | 13.97,9.21 15.05,9.21 v15.62,9.78 | C2.1 13.97,9.21
  other vias: 13.97,9.27
  pour Horz (isolate 0.152, rank 3): 0,30.48 30.48,30.48 30.48,0 0,0
5V  (via drill 0.3)
  Top 0.457: D2.A 11.42,10.54 v10.29,10.54 | JP2.3 JP2.1
  Top 0.559: JP2.3 1.85,5.77 3.73,5.77 4.93,4.57 v6.73,4.57 | J5.VBUS1 17.87,6.77 v17.02,7.62 | J5.VBUS2 22.77,6.95 v22.73,6.99
  Bottom 0.559: 6.73,6.86 v6.73,4.57 v5.84,4.57 v4.95,4.57 | 6.73,6.86 6.73,7.24 6.99,7.5 D1.C 9.06,7.5 U2.4 9.49,7.65 10.1,8.26 10.1,9.89 10.29,10.08 v10.29,10.54 | C3.1 6.73,6.86
  pour Horz (isolate 0.152, rank 2): 0,7.62 24.13,7.62 24.13,3.81 0,3.81
!POWER_LOSS!
  Top 0.152: U8.D3 21.96,27.4 U1.2
ARTEMIS_!RESET  (via drill 0.3)
  Top 0.152: v8.13,23.62 7.75,23.24 7.75,20.45 J14.10 5.97,18.67 4.57,18.67 4.19,19.05 4.19,25.02 6.35,27.18 J7.1 | v13.84,25.37 13.88,25.4 15.56,25.4 16.57,24.39 17.4,24.39 18.18,25.18 18.18,25.4 | S3.4 27.14,19.01 27.43,19.3 28.57,19.3 28.85,19.58 28.85,20.29 28.34,20.8 27.59,20.8 27.14,21.25 S3.3 27.12,22.35 26.29,22.35 25.15,23.5 21.84,23.5 20.52,24.82 20.52,25.08 20.19,25.4 U8.~RST 18.18,25.4 | v18.18,26.29 18.18,25.4 | v21.34,9.53 20.68,8.87 v19.81,8.87
  Bottom 0.152: C44.1 R28.1 19.81,7.87 19.81,8.13 | v13.84,25.37 13.11,25.37 13.05,25.43 9.93,25.43 v8.13,23.62 | v21.34,9.53 21.16,9.7 21.16,12.88 20.04,14 20.04,17.41 20.32,17.69 20.32,18.63 20.04,18.91 20.04,21.16 19.36,21.84 19.36,25.11 v18.18,26.29 | 19.81,8.13 v19.81,8.87 | C42.2 19.81,8.12 19.81,8.13
ARTEMIS_!RTS!
  Bottom 0.152: U10.4 23.25,2.04 23.88,2.67 23.88,5.97 23.49,6.36 22.35,6.36 C43.1 C42.1
ARTEMIS_BOOT  (via drill 0.3)
  Top 0.152: v16.26,26.39 16,26.65 12.37,26.65 12.12,26.9 U8.BOOT 10.14,26.9 9.53,26.29 R29.2
  Bottom 0.152: v16.26,26.39 16.59,26.06 16.86,26.06 17.09,25.83 17.45,25.83 18.75,24.54 18.75,21.59 19.43,20.91 19.43,18.66 19.71,18.38 19.71,17.94 19.43,17.66 19.43,10.12 21.07,8.48 21.23,8.48 C43.2
ARTEMIS_RX0  (via drill 0.3)
  Top 0.152: v17.53,13.59 17.27,13.59 16.51,12.83 D11.C | U8.RXI-0 11.87,28.9 12.83,27.94 15.88,27.94 17.4,26.42 17.4,25.15 v17.18,24.92
  Bottom 0.152: U10.8 16.64,2.54 14.73,4.45 14.73,8.05 17.8,11.12 17.8,13.3 v17.53,13.58 v17.53,13.59 17.53,16 18.19,16.66 18.19,17.75 18.14,17.8 18.14,24 17.22,24.92 v17.18,24.92
ARTEMIS_SWDCK  (via drill 0.3)
  Top 0.152: U8.SWDCK 10.1,29.4 9.65,28.96 v9.65,27.69
  Bottom 0.152: J14.4 7,23.5 7.71,24.21 7.71,27.4 8,27.69 v9.65,27.69
ARTEMIS_SWDIO
  Top 0.152: J14.2 7.62,25.4 U8.SWDIO
ARTEMIS_TX0  (via drill 0.3)
  Top 0.152: U8.TXO-0 15.84,25.9 16.04,25.71 16.46,25.71 v16.64,25.53 | v18.01,10.16 18.66,10.16 D12.C
  Bottom 0.152: U10.9 16.57,3.04 15.04,4.57 15.04,7.84 17.05,9.86 17.7,9.86 v18.01,10.16 18.01,10.9 18.11,11 18.11,16.16 18.49,16.54 18.49,17.88 18.47,17.91 18.47,20.19 18.44,20.22 18.44,24.41 17.32,25.53 v16.64,25.53
ARTEMIS_~AD11
  Top 0.152: U8.~AD11 16.24,18.2 14.57,16.52 13.4,16.52 12.83,15.95 9.05,15.95 7.83,14.73 4.06,14.73 1.27,11.94 J4.1
ARTEMIS_~AD12/TX1
  Top 0.152: U8.~AD12 13.24,18.32 11.81,16.89 4.05,16.89 3.65,16.49 1.29,16.49 J4.3
ARTEMIS_~AD13/RX1
  Top 0.152: J4.2 1.65,13.97 4.27,16.59 12.25,16.59 13.04,17.37 13.94,17.37 14.25,17.69 14.25,18.13 14.24,18.14 U8.~AD13
ARTEMIS_~AD32  (via drill 0.3)
  Top 0.152: U8.~AD32 12.24,17.95 11.89,17.6 7.4,17.6 v7.3,17.5
  Bottom 0.152: v7.3,17.5 4.72,17.5 3.17,19.05 J4.4
CC3
  Top 0.152: R26.2 24.9,7.6 24.9,6.98 25.53,6.35 25.53,4.7 24.51,3.68 22.73,3.68 22.07,4.35 J5.B5
CC4
  Top 0.152: R27.2 14.74,4.56 16.32,2.98 18.22,2.98 19.07,3.83 J5.A5
CHG_LED
  Bottom 0.152: R5.1 12.7,10.45 12.22,9.97 10.89,9.97 10.63,9.71 10.63,8.37 10.61,8.35 10.61,6.67 11.11,6.16 U2.1
D+2  (via drill 0.3)
  Top 0.152: v21.08,3.68 21.07,3.69 21.07,5.08 | J5.B6 21.07,5.08 | J5.A6 20.07,5.2 20.19,5.08 21.07,5.08
  Bottom 0.152: U10.1 21.23,3.54 v21.08,3.68
D-2  (via drill 0.3)
  Top 0.152: J5.A7 20.57,6.74 20.45,6.86 19.68,6.86 19.56,6.73 19.56,6.02 J5.B7 19.57,3.92 v20.32,3.17
  Bottom 0.152: U10.2 20.45,3.04 v20.32,3.17
DAT1  (via drill 0.3)
  Top 0.152: U8.~D26 13.74,17.93 v13.72,17.91
  Vertical 0.152: v13.72,17.91 10.63,20.99 9.74,20.99 8.64,22.1 v8.64,22.56
  Bottom 0.152: v8.64,22.56 8.64,23.11 8.92,23.4 J6.RSV2
DAT2  (via drill 0.3)
  Top 0.152: U8.~D4 15.65,22.9 v16.86,21.69
  Bottom 0.152: v16.86,21.69 16.86,22.19 17.2,22.53 J6.RSV1
GND  (via drill 0.3)
  Top 0.203: C7.2 24.27,13.84 25.4,13.84 25.78,14.22 25.78,15.49 25.65,15.62 U4.2
  Top 0.457: U4.2 24.26,15.62 v23.88,16
  Bottom 0.152: U13.20 27.27,16.67 | 27.05,17.27 v26.54,17.27 27.3,17.27 27.8,16.78 U13.18 28.24,16.76 v28.96,16.76
  other vias: 9.78,18.54 12.32,22.1 16.51,15.24 17.65,17.4 17.53,22.1 13.84,29.08 8.89,29.08 6.35,26.16 13.34,13.84 7.75,10.16 10.16,6.35 11.56,3.81 12.7,5.08 3.3,6.99 21.34,2.03 17.02,8.76 25.78,7.49 16.51,6.99 18.03,27.69 22.61,24.38 26.12,24.13 21.97,15.62 20.7,19.3 17.02,28.96 23.5,22.86 20.57,23.24 24.13,10.16 22.86,7.75 22.61,10.03 29.84,6.99 8.51,24.77 3.05,17.65 5.33,0.89
  pour Top (isolate 0.152, rank 6): 0,0 0,30.48 30.48,30.48 30.48,0
  pour Bottom (isolate 0.152, rank 6): 30.48,0 30.48,30.48 0,30.48 0,0
  pour Vertical (isolate 0.152): 0,30.48 30.48,30.48 30.48,0 0,0
ICM-20948-LV_!CS!
  Bottom 0.152: U13.22 26.47,15.82 26.67,15.62 28.19,15.62 28.71,15.11 R46.1 Q9.2
ICM-20948-LV_#_1.8V  (via drill 0.3)
  Top 0.152: v26.93,14.74 26.93,15.12 27.56,15.75 v28.83,15.75 | v28.32,20.07 27.73,20.07 25.7,22.1 v24.14,22.1
  Bottom 0.152: Q9.1 R46.2 29.71,14.99 28.95,15.75 v28.83,15.75 29.84,16.76 29.84,18.8 | Q7.1 28.31,22.52 28.31,21.08 R44.2 28.44,20.18 v28.32,20.07 28.96,20.07 29.84,19.18 29.84,18.8 | Q10.1 24.39,22.35 v24.14,22.1 R48.2 25.65,20.58 25.65,19.94 | C52.1 24.28,9.54 U14.5 25.84,11.49 | 25.84,11.49 26.17,11.82 Q1.1 R40.2 26.93,14.73 v26.93,14.74 | C53.1 24.64,18.79 24.64,19 25.58,19.94 25.65,19.94 | U13.8 26.07,19.72 25.85,19.94 25.65,19.94 | R41.2 Q3.1 24.23,11.93 24.45,11.93 24.89,11.49 25.84,11.49 | U13.13 29.83,18.78 29.84,18.8
ICM-20948-LV_INT
  Bottom 0.152: U13.12 27.67,20.84 27.56,20.95 R44.1 Q7.2
ICM-20948-LV_MISO
  Bottom 0.152: U13.9 26.47,20.39 25.9,20.96 R48.1 25.39,21.84 Q10.2
ICM-20948-LV_MOSI
  Bottom 0.152: U13.24 25.67,15 R41.1 | R41.1 | Q3.2 R41.1
ICM-20948-LV_SCK
  Bottom 0.152: Q1.2 R40.1 27.17,14.22 27.46,14.52 27.46,14.96 27.1,15.32 26.47,15.32 26.07,15.71 U13.23
ICM_!CS!  (via drill 0.3)
  Top 0.152: v29.59,25.06 29.59,24.68 29.76,24.5 29.76,17.9 29.49,17.63 29.49,15.65 29.05,15.21 28.14,15.21 27.81,14.89 27.81,13.34 v28.07,13.08 | U8.~D44 20.45,29.4 21.2,28.64 22.53,28.64 23.37,29.48 v23.37,29.59
  Bottom 0.152: Q9.3 29.21,11.05 | 29.21,11.05 29.21,10.66 R47.1 | v28.07,13.08 28.07,11.37 28.39,11.05 29.21,11.05 | v23.37,29.59 23.51,29.74 24.47,29.74 24.99,29.22 24.99,26.7 26.19,25.5 26.41,25.5 26.85,25.06 v29.59,25.06
ICM_INT  (via drill 0.3)
  Top 0.152: v24.25,29.2 24,28.95 23.27,28.95 22.66,28.34 21.07,28.34 20.5,28.9 U8.~D37
  Bottom 0.152: v24.25,29.2 24.55,28.9 24.55,26.67 26.03,25.2 26.28,25.2 26.79,24.69 28.87,24.69 29.03,24.52 29.73,24.52 29.87,24.39 29.87,23.14 29.73,23 R45.1 28.97,23 28.77,23.2 28.74,23.2 28.57,23.37 28.57,23.62 28.4,23.8 Q7.3
ICM_PWR  (via drill 0.3)
  Top 0.152: v26.16,5.46 26.16,4.9 23.9,2.64 16.05,2.64 14.25,4.45 8.14,4.45 v8.14,4.43 | U8.~D27 10.11,20.9 9.76,20.55 v9.76,20.04
  Vertical 0.152: v8.14,4.43 6.96,5.6 6.96,11.02 7.83,11.89 7.83,17.36 9.76,19.29 v9.76,20.04
  Bottom 0.152: v26.16,5.46 27.13,5.46 27.5,5.83 U14.3
MICROSD_!CS!  (via drill 0.3)
  Top 0.152: v15.11,21.97 14.72,21.97 14.19,22.5 13.62,22.5 12.52,21.4 U8.~D23
  Bottom 0.152: v15.11,21.97 15.88,21.97 16.09,22.19 J6.CS
MICROSD_PWR
  Top 0.152: Q2.1 5.38,16.26 12.57,16.26 13.26,16.94 14.19,16.94 14.74,17.49 U8.D15
MISO  (via drill 0.3)
  Top 0.152: U8.~D6 11.74,18.34 11.3,17.91 8.38,17.91 8,18.29 v8,18.67 8,20.27 8.05,20.32 8.05,21.46 8.49,21.9 v9.97,21.9 U8.~D22
  Bottom 0.152: Q10.3 24.89,24.39 R49.1 23.62,24.89 23.05,25.46 23.05,28.26 22.62,28.68 20.93,28.68 20.57,28.32 7.49,28.32 4.19,25.02 4.19,18.92 5.31,17.8 6.72,17.8 6.95,18.03 7.37,18.03 v8,18.67 | v9.97,21.9 10.6,22.53 J6.DO
MOSI  (via drill 0.3)
  Top 0.152: v15.49,24.64 14.76,23.9 U8.D7
  Bottom 0.152: J6.DI 14.99,24.14 v15.49,24.64 15.49,26.68 15.21,26.96 15.21,27.4 15.53,27.71 16.12,27.71 17.01,26.82 19.23,26.82 19.66,26.39 19.66,21.97 20.27,21.36 21.7,21.36 22.68,20.38 22.68,15.04 23.1,14.62 23.1,11.82 23.55,11.38 Q3.3
N$1
  Top 0.305: BT1.+ 23,21.84 24.52,20.32 D3.A R1.1
N$7
  Bottom 0.152: R4.2 12.7,7.37 12.42,7.65 U2.5
N$11  (via drill 0.3)
  Top 0.152: D2.C 10.94,11.81 v10.16,11.81
  Bottom 0.152: v10.16,11.81 12.59,11.81 R5.2
N$20
  Top 0.152: U8.XO 17.24,18.38 15.26,16.4 15.26,15.62 | Y3.P$2 15.26,15.62 | C29.2 15.14,15.74 15.26,15.62
N$21
  Top 0.152: Y3.P$1 17.74,15.26 17.74,15.49 17.78,15.53 17.78,15.62 | U8.XI 17.74,18.37 17.12,17.75 17.12,17.17 17.78,16.51 17.78,15.62 | C30.2 17.79,15.61 17.78,15.62
N$24  (via drill 0.3)
  Top 0.152: v14.61,13.72 14.61,12.91 14.7,12.81 14.7,11.28 LED1.A
  Bottom 0.152: R22.1 14.8,12.37 14.8,12.45 14.61,12.65 v14.61,13.72
N$25  (via drill 0.3)
  Top 0.152: v21.46,13.34 21.46,12.43 D9.A
  Bottom 0.152: R23.1 21.46,11.56 v21.46,13.34
N$26  (via drill 0.3)
  Top 0.152: D12.A 19.44,12.7 v20.45,12.7
  Bottom 0.152: v20.45,12.7 20.45,12.06 R25.1
N$27  (via drill 0.3)
  Top 0.152: D11.A 16.51,10.66 17.14,10.66 17.27,10.79 v17.27,11.43
  Bottom 0.152: v17.27,11.43 17.02,11.43 R24.1
N$30
  Bottom 0.152: C51.1 26.54,22.23 26.54,20.75 26.87,20.42 U13.10
PWR_LED  (via drill 0.3)
  Top 0.152: v16.76,20.7 16.76,18.92 U8.~AD29
  Bottom 0.152: v16.76,20.7 16.76,17.27 13.95,14.45 13.95,12.6 14.08,12.46 14.37,12.46 14.5,12.32 14.5,11.67 R22.2
QWIIC_3.3V
  Top 0.559: U4.5 22.32,14 22.61,13.72 22.61,12.32 22.98,11.95 C7.1 C5.1 23.38,10.92 J11.2
QWIIC_PWR
  Top 0.152: U8.~D18 21.5,20.9 22.12,20.29 22.12,19.3 | 22.12,19.3 22.12,18.01 23.56,16.57 U4.3 | R3.2 22.1,19.32 22.12,19.3
SCK  (via drill 0.3)
  Top 0.152: v12.7,24.89 12.21,24.4 U8.~D5 | v13.08,8.28 12.83,8.53 12.83,12.83 12.37,13.28 10.92,13.28 10.03,14.17 v10.03,14.86
  Bottom 0.152: v12.7,24.89 12.79,24.8 J6.SCLK 12.92,23.27 12.92,21.96 13.46,21.42 15.15,21.42 15.55,21.02 15.55,20.13 15.11,19.68 12.8,19.68 10.03,16.92 v10.03,14.86 | v13.08,8.28 13.08,7.94 14.3,6.72 14.3,4.45 17.11,1.64 17.11,1.18 17.38,0.91 23.26,0.91 23.62,1.27 23.62,1.85 24.64,2.87 24.64,3.52 25.4,4.29 25.4,6.35 26.67,7.62 Q1.3
SCL  (via drill 0.3)
  Top 0.152: U8.D8 11.95,24.9 12.48,25.43 12.93,25.43 13.52,24.83 14.34,24.83 v14.36,24.81 | J11.4 25.4,13.34 26.16,14.1 26.16,16.66 24.88,17.94 v23.37,17.94
  Bottom 0.152: v14.36,24.81 14.48,24.92 14.48,27.09 15.4,28.02 16.25,28.02 17.14,27.13 19.35,27.13 19.96,26.52 19.96,22.2 20.45,21.72 21.84,21.72 22.99,20.57 22.99,18.03 23.08,17.94 v23.37,17.94
SD_PWR  (via drill 0.3)
  Top 0.305: v12.44,20.58 12.44,20.71 13.7,21.97 v13.97,21.97 | v6.48,18.41 5.67,17.61 Q2.3 | C46.1 v8.89,20.7
  Bottom 0.305: v13.97,21.97 13.89,22.05 J6.VCC | v6.48,18.41 6.76,18.7 7.16,18.7 8,19.54 8,20.32 8.38,20.7 v8.89,20.7 8.9,20.69 12.34,20.69 v12.44,20.58
SDA  (via drill 0.3)
  Top 0.152: U8.D9 15.53,27.4 v15.75,27.18 | v22.48,9.14 26.04,9.14 26.67,9.78 26.67,11.56 26.3,11.93 J11.3
  Bottom 0.152: v15.75,27.18 16.22,27.18 17.27,26.14 17.58,26.14 17.96,25.75 18.19,25.75 19.05,24.89 19.05,21.72 19.74,21.03 19.74,18.79 20.02,18.51 20.02,17.81 19.74,17.53 19.74,10.24 21.09,8.89 22.23,8.89 v22.48,9.14
STATLED  (via drill 0.3)
  Top 0.152: v21.33,20.32 21.25,20.4 U8.~D19
  Bottom 0.152: R23.2 22.1,13.59 21.33,14.36 v21.33,20.32
SWO  (via drill 0.3)
  Top 0.152: U8.~AD33/SWO 15.24,20.34 14.87,20.7 v14.73,20.7
  Bottom 0.152: v14.73,20.7 13.9,20.7 13.49,21.12 12.96,21.12 12.94,21.13 9.22,21.13 8.13,22.23 J14.6
V_BATT  (via drill 0.3)
  Top 0.152: J2.2 9.16,6.49 9.02,6.35
  Top 0.559: 9.02,6.35 v8.13,6.35 v7.49,6.35
  Bottom 0.152: D1.A
  Bottom 0.305: U2.3 9.21,3.81 | 9.21,3.81 9.21,1.59 J1.1 | C4.1 9.21,3.81 | U2.3 8.29,5.05 8.13,5.21 D1.A | U2.3 9.21,6.03 8.89,6.35 v8.13,6.35 v7.49,6.35
VCC_1  (via drill 0.3)
  Top 0.305: R1.2 25.54,19.31 25.47,19.39 24.28,19.39 v24.23,19.43 23.87,19.43 23.77,19.53 23.62,19.53 | D3.C 22.73,19.43 | 22.73,19.43 D6.C | C32.1 20.57,16.51 20.45,16.63 C33.1 C31.2 19.55,17.94 19.33,18.16 v19.18,18.16 18.97,18.16 18.74,18.39 U8.VDD@37 18.74,19.41 18.45,19.7 U8.VDD@36 18.24,20.37 v17.53,21.08 | 23.62,19.53 23.27,19.53 23.17,19.43 22.73,19.43 | v23.6,20.07 23.6,19.55 23.62,19.53
  Horz 0.305: 23.6,19.68 23.62,19.65
  Horz 0.559: v24.23,19.43 24.23,19.5 24.08,19.65 23.62,19.65 23.21,19.65 21.72,18.16 v19.18,18.16 17.53,19.81 v17.53,21.08 | v23.6,20.07 23.6,19.68
  Bottom 0.152: R28.2 19.05,10.31 19,10.36 19,17.98 v19.18,18.16
VIN  (via drill 0.3)
  Top 0.152: JP2.4 4.95,8.89 5.08,8.76 R2.2
  Top 0.457: JP2.2 JP2.4 | v23.36,15.36 23.36,15.23 v23.86,14.73
  Top 0.559: U4.1 23.92,14.67 v23.86,14.73
  Horz 0.559: v23.86,14.73 23.86,14.69
  Bottom 0.457: R7.2 4.33,14.48 3.05,13.2 3.05,8.89
  Bottom 0.559: JP2.4 3.05,8.89 4.41,8.89 4.51,8.79 | 4.51,8.79 4.45,8.79 C1.1 | 4.51,8.79 7.39,8.79 v7.75,9.14 7.75,9.17 8.05,9.17 8.09,9.21 U3.1
  pour Horz (isolate 0.152): 0,7.62 8.89,7.62 15.24,13.97 25.4,13.97 25.4,16.51 12.7,16.51 6.35,10.16 0,10.16
VIN/3  (via drill 0.3)
  Top 0.152: U8.AD34 15.27,18.43 v15.27,18.03
  Bottom 0.152: v15.27,18.03 11.46,14.22 5.71,14.22 R7.1 4.95,14.98 4.95,16.26 R6.2
VREG_EN
  Top 0.152: J3.1 6.21,12.7 6.81,12.11 6.81,11.05 | R2.1 5.85,7.12 6.81,8.08 6.81,11.05 | VE.2 6.83,11.02 6.81,11.05
  Bottom 0.152: U3.3 7.81,11.11 6.22,12.7 J3.1
VREG_EN1  (via drill 0.3)
  Top 0.152: U8.~D25 12.74,20.06 v13.27,20.58 | v8.97,14.86 8.97,13.93 8.89,13.84 VE.1
  Bottom 0.152: v8.97,14.86 8.97,16.29 v13.27,20.58

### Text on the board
Bottom: v10
Measures: Units in inches
tDocu: 4-layer board | 1.6mm thickness | ENIG finish | N. Seidle

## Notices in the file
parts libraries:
SparkFun-Aesthetics: Licensing: Creative Commons ShareAlike 4.0 International - https://creativecommons.org/licenses/by-sa/4.0
SparkFun-Aesthetics: Released under the Creative Commons Attribution Share-Alike 4.0 License
SparkFun-Aesthetics: https://creativecommons.org/licenses/by-sa/4.0
